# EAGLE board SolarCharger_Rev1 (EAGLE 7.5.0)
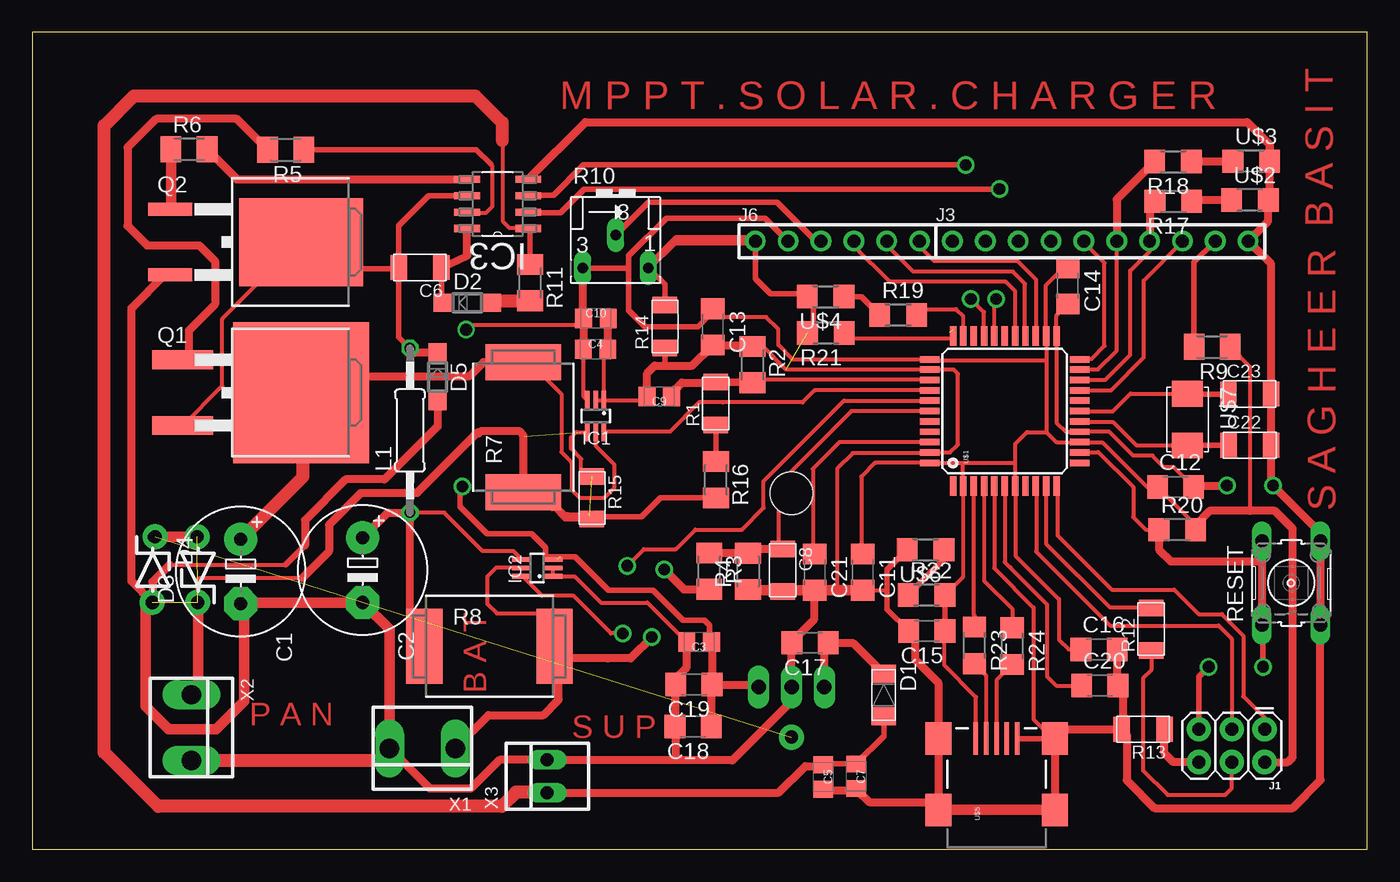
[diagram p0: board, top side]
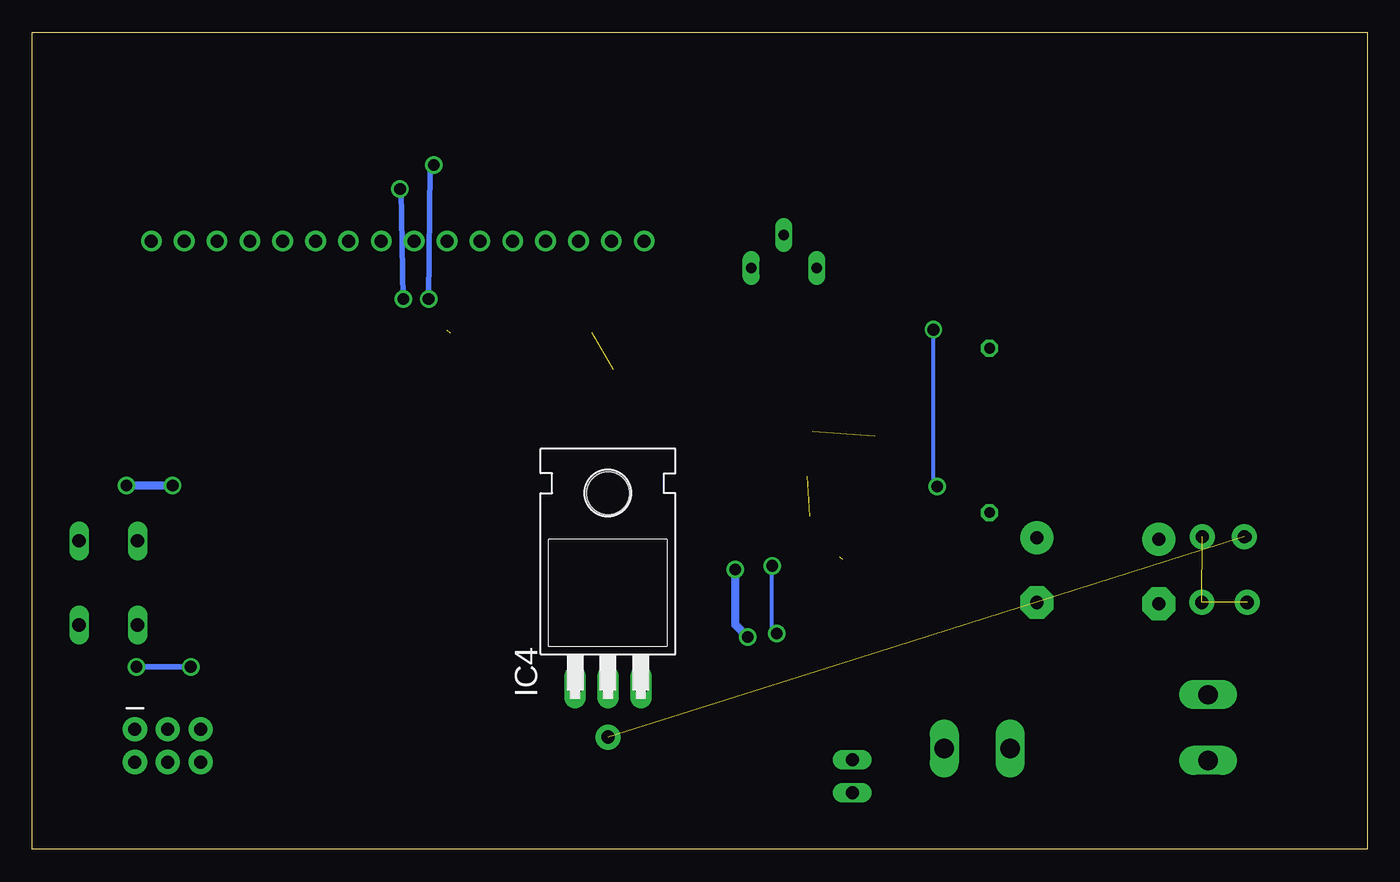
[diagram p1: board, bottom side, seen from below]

Size 103.17 x 63.12 mm. Coordinates in mm from the lower left corner, seen from the top.
Outline: 0,0 103.17,0 103.17,63.12 0,63.12 0,0
Copper layers (1*16): Top 0.035mm / dielectric 1.5mm / Bottom 0.035mm
Design rules "default": minimum track width 10mil, minimum drill 24mil, track to track 8mil, track to pad 8mil, pad to pad 8mil, via to via 8mil, smd to smd 8mil, copper to edge 40mil, drill to drill 8mil, minimum pad ring 10mil, minimum via ring 8mil, stop-mask expansion 4mil, vias tented up to drill 0mil, thermal gap 10mil

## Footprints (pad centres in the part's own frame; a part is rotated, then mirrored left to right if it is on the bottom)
10MM = drill 1.016 pad 2.54: + -2.5,0 | drill 1.016 pad 2.54 octagon: - 2.5,0
C0805 = smd 1.3 x 1.5: 1 -0.95,0; 2 0.95,0
C1206FAB = smd 1.27 x 1.905: 1 -1.651,0; 2 1.651,0
C1206 = smd 1.6 x 1.8: 1 -1.4,0; 2 1.4,0
MINI-SMA = smd 1.4 x 1.9: ANODE 1.65,0; KATHODE -1.65,0
SOD123 = smd 1.4 x 1.4: A 1.9,0; C -1.9,0
ZDIO-5 = drill 0.813 octagon: A 2.54,0; C -2.54,0
SC70-6_LONG = smd 0.35 x 1.5: 1 -0.65,-1.2; 2 0,-1.2; 3 0.65,-1.2; 4 0.65,1.2; 5 0,1.2; 6 -0.65,1.2
SOIC8 = smd 1.981 x 0.559: 1 -2.362,1.905; 2 -2.362,0.635; 3 -2.362,-0.635; 4 -2.362,-1.905; 5 2.362,-1.905; 6 2.362,-0.635; 7 2.362,0.635; 8 2.362,1.905
TO220H = drill 1.118 long: 1 -2.54,-10.16; 2 0,-10.16; 3 2.54,-10.16 | hole 3.302: 0,4.826
2X3 = drill 1.016 pad 1.88: 1 0,0; 2 0,2.54; 3 2.54,0; 4 2.54,2.54; 5 5.08,0; 6 5.08,2.54
100MIL_10X_ROUND = drill 1 pad 1.6: 1 -8.89,0; 2 -6.35,0; 3 -3.81,0; 4 -1.27,0; 5 1.27,0; 6 3.81,0; 7 6.35,0; 8 8.89,0; 9 11.43,0; 10 13.97,0
100MIL_6X_ROUND = drill 1 pad 1.6: 1 -6.35,0; 2 -3.81,0; 3 -1.27,0; 4 1.27,0; 5 3.81,0; 6 6.35,0
0207/12 = drill 0.813 octagon: 1 -6.35,0; 2 6.35,0
TO263-3 = smd 1.45 x 4.7: 1 -2.54,-5.65; 3 2.54,-5.65 | smd 10.9 x 10.5: TAB 0,3.5
TO263-3@1 = smd 1 x 3.4: 1 -2.54,-6.6; 3 2.54,-6.6 | smd 6.8 x 9.6: TAB 0,3.5
R1206FAB = smd 1.27 x 1.905: 1 -1.651,0; 2 1.651,0
M1206 = smd 1.6 x 2: 1 -1.4,0; 2 1.4,0
SMR = smd 2.8 x 5.8: 1 5.029,0; 2 -5.029,0
B25X = drill 0.813 long: A 2.54,-1.905; E -2.54,-1.905; S 0,0.635
R1206 = smd 1.6 x 1.803: 1 -1.422,0; 2 1.422,0
B3F-10XX = drill 1.016 long: 1 -3.251,2.261; 2 3.251,2.261; 3 -3.251,-2.261; 4 3.251,-2.261
SPARKFUN-DIGITALIC_TQFP44 = smd 1.5 x 0.5: 1 -5.8,4; 2 -5.8,3.2; 3 -5.8,2.4; 4 -5.8,1.6; 5 -5.8,0.8; 6 -5.8,0; 7 -5.8,-0.8; 8 -5.8,-1.6; 9 -5.8,-2.4; 10 -5.8,-3.2; 11 -5.8,-4; 23 5.8,-4; 24 5.8,-3.2; 25 5.8,-2.4; 26 5.8,-1.6; 27 5.8,-0.8; 28 5.8,0; 29 5.8,0.8; 30 5.8,1.6; 31 5.8,2.4; 32 5.8,3.2; 33 5.8,4 | smd 0.5 x 1.5: 12 -4,-5.8; 13 -3.2,-5.8; 14 -2.4,-5.8; 15 -1.6,-5.8; 16 -0.8,-5.8; 17 0,-5.8; 18 0.8,-5.8; 19 1.6,-5.8; 20 2.4,-5.8; 21 3.2,-5.8; 22 4,-5.8; 34 4,5.8; 35 3.2,5.8; 36 2.4,5.8; 37 1.6,5.8; 38 0.8,5.8; 39 0,5.8; 40 -0.8,5.8; 41 -1.6,5.8; 42 -2.4,5.8; 43 -3.2,5.8; 44 -4,5.8
LED1206 = smd 1.6 x 1.803: 1 -1.422,0; 2 1.422,0
USB_MINIB = smd 2.5 x 0.35: D+ 3.77,0; D- 3.77,0.8; GND 3.77,-1.6; ID 3.77,-0.8; VBUS 3.77,1.6 | smd 2.5 x 2: SHIELD@1 -1.73,-4.5; SHIELD@2 -1.73,4.5; SHIELD@3 3.77,4.5; SHIELD@4 3.77,-4.5
2-SMD-5X3MM = smd 2 x 2.4: P$1 -2,0; P$2 2,0
200MIL_2X = drill 1.5 long: 1 -2.54,0; 2 2.54,0
22-23-2021 = drill 1 long: 1 -1.27,0; 2 1.27,0

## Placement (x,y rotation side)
C1  680u  [10MM]  16.1,21.46 270 top
C2  820u  [10MM]  25.53,21.56 270 top
C3  100n  [C0805]  51.54,16 180 top
C4  100n  [C0805]  43.54,38.63 0 top
C5  100n  [C0805]  61.14,5.59 270 top
C6  100n  [C1206FAB]  29.97,44.94 180 top
C7  1u  [C0805]  63.68,5.64 270 top
C8  100n  [C1206FAB]  57.99,21.56 270 top
C9  100n  [C0805]  48.46,34.98 180 top
C10  100n  [C0805]  43.56,41.02 0 top
C11  0.1u  [C1206]  64.19,21.41 270 top
C12  0.1u  [C1206]  88.37,27.99 0 top
C13  0.1u  [C1206]  52.6,40.36 270 top
C14  0.1u  [C1206]  80.04,43.54 270 top
C15  0.1u  [C1206]  69.14,16.87 180 top
C16  0.1u  [C1206]  82.45,15.44 0 top
C17  470u  [C1206]  60.12,15.95 180 top
C18  1uf  [C1206]  51.08,9.47 180 top
C19  0.1u  [C1206]  51.13,12.73 180 top
C20  0.1u  [C1206]  82.5,12.65 0 top
C21  0.1u  [C1206]  60.48,21.41 270 top
C22  18pF  [C1206FAB]  94.11,31.22 0 top
C23  18pF  [C1206FAB]  94.1,35.17 0 top
D1  CDBM1100-G  [MINI-SMA]  65.81,11.91 270 top
D2  SCHOTTKYSOD123  [SOD123]  33.62,42.23 0 top
D3  15V  [ZDIO-5]  12.8,21.59 90 top
D4  5V  [ZDIO-5]  9.32,21.59 270 top
D5  SCHOTTKYSOD123  [SOD123]  31.33,36.5 270 top
IC1  INA213LONG  [SC70-6_LONG]  43.54,33.48 180 top
IC2  INA213LONG  [SC70-6_LONG]  39.01,21.74 90 top
IC3  IR2104  [SOIC8]  35.97,49.86 180 top
IC4  7805T  [TO220H]  58.68,22.69 0 bottom
J1  FEMALE 2x3  [2X3]  95.25,9.27 180 top
J3  Digital2  [100MIL_10X_ROUND]  80.01,46.99 0 top
J6  Analog  [100MIL_6X_ROUND]  62.23,46.99 0 top
L1  100u  [0207/12]  29.18,32.36 90 top
Q1  IPB136N08N3  [TO263-3]  17.27,35.28 270 top
Q2  IPB136N08N3  [TO263-3@1]  17.27,46.91 270 top
R1  6k  [R1206FAB]  52.83,34.44 90 top
R2  10k  [M1206]  55.68,37.44 270 top
R3  22k  [M1206]  52.32,21.49 270 top
R4  10k  [M1206]  55.32,21.46 90 top
R5  10  [M1206]  19.58,54.05 180 top
R6  10  [M1206]  12.12,54.08 0 top
R7  shunt 1  [SMR]  37.95,32.6 90 top
R8  shunt 2  [SMR]  35.33,15.69 0 top
R9  220  [M1206]  91.19,38.81 180 top
R10  10k  [B25X]  45.09,46.81 0 top
R11  10  [M1206]  38.48,43.77 270 top
R12  0  [R1206FAB]  86.48,17 90 top
R13  0  [R1206FAB]  85.85,9.27 180 top
R14  0  [R1206FAB]  48.9,40.39 90 top
R15  0  [R1206FAB]  43.26,27.15 270 top
R16  33k  [M1206]  52.83,28.55 270 top
R17  499  [R1206]  88.19,50.06 180 top
R18  499  [R1206]  88.16,53.14 180 top
R19  499  [R1206]  66.93,41.27 0 top
R20  10k  [R1206]  88.49,24.69 0 top
R21  680  [R1206]  61.34,39.9 180 top
R22  499  [R1206]  69.11,19.63 0 top
R23  22  [R1206]  72.82,15.75 270 top
R24  22  [R1206]  75.74,15.7 270 top
RESET  [B3F-10XX]  97.31,20.57 90 top
U$1  ATMEGA32U4TQFP  [SPARKFUN-DIGITALIC_TQFP44]  75.16,33.86 90 top
U$2  LED  [LED1206]  94.11,50.16 0 top
U$3  LED  [LED1206]  94.21,53.16 0 top
U$4  LED  [LED1206]  61.32,42.7 180 top
U$5  USB_MINIB  [USB_MINIB]  74.52,4.78 90 top
U$6  LED  [LED1206]  69.04,23.14 180 top
U$7  CRYSTAL  [2-SMD-5X3MM]  89.28,33.2 270 top
X1  Battery  [200MIL_2X]  30.15,7.8 180 top
X2  Pannel  [200MIL_2X]  12.29,9.4 270 top
X3  Supply  [22-23-2021]  39.8,5.64 90 top

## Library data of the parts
C1-C5 C7 C9 C10 = 00Capacitor
C6 C8 C22 C23 D1 R1 R12-R15 R17-R24 U$2-U$7 = fab
C11-C21 L1 R2-R6 R9 R11 R16 = rcl
D2 D5 = 00Diode
D3 D4 = diode
IC1 IC2 = 00Sensor; GAIN: 50
IC3 = 00Logic
IC4 = linear
J1 = SparkFun-Connectors; PROD_ID: CONN-11566
J3 J6 X1 X2 = 00Connector
Q1 Q2 = 00Mosfet
R7 R8 = resistor-shunt; OC_FARNELL: unknown; OC_NEWARK: unknown
R10 = pot
RESET = switch-omron; MPN: B3F-1000; OC_FARNELL: 176432; OC_NEWARK: 36M3542
U$1 = SparkFun-Retired; PROD_ID: IC-11161
X3 = 00Connector; MF: MOLEX; MPN: 22-23-2021; OC_FARNELL: 1462926; OC_NEWARK: 25C3832

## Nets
!SD!: IC3.3 U$1.30
+5V: C3.1 C4.1 C10.1 C11.1 C12.1 C13.1 C14.1 C15.1 C16.1 C18.1 C19.1 IC1.3 IC2.3 IC4.3 J1.2 J6.2 R9.1 R10.E R20.2 R22.2 U$1.2 U$1.7 U$1.14 U$1.24 U$1.34 U$1.44 U$5.VBUS
+12V: C5.1 C7.1 D1.ANODE IC3.1 R11.1 X3.1
AREF: C21.1 U$1.42
BATTERY: IC2.5 R3.2 R8.1 X1.1
D4: J3.5 U$1.22
D5: J3.6 R18.2 U$1.21
D6: J3.7 R17.2 U$1.20
D7: J3.8 U$1.19
D13: R19.2 U$1.32
D+: R24.1 U$1.4
D-: R23.1 U$1.3
E: J6.6 U$1.25
GND: C1.- C2.- C3.2 C4.2 C5.2 C7.2 C8.2 C9.2 C10.2 C11.2 C12.2 C13.2 C14.2 C15.2 C16.2 C17.2 C18.2 C19.2 C20.2 C21.2 C22.2 C23.2 D4.A D5.A IC1.1 IC1.2 IC2.1 IC2.2 IC3.4 IC4.2 J3.10 J6.1 Q2.3 R2.1 R4.1 R13.2 R14.1 R21.2 RESET.3 RESET.4 U$1.5 U$1.15 U$1.23 U$1.35 U$1.43 U$2.2 U$3.2 U$4.2 U$5.GND U$5.SHIELD@1 U$5.SHIELD@2 U$5.SHIELD@3 U$5.SHIELD@4 U$6.2 X1.2 X2.2 X3.2
IIN_SENSE: IC1.6 U$1.37
IOUT_SENSE: IC2.6 U$1.38
MISO: J1.1 U$1.11
MOSI: R12.2 U$1.10
N$1: J1.4 R12.1
N$2: J1.6 R13.1
N$3: R10.A R14.2
N$4: Q1.1 R5.2
N$5: R15.1 R16.2
N$7: Q2.1 R6.1
N$9: J3.9 R9.2
N$10: J6.3 R10.S
N$11: D2.A R11.2
N$12: C6.1 D2.C IC3.8
N$14: IC3.7 R5.1
N$15: IC3.5 R6.2
N$17: R1.1 R16.1
N$19: D3.A D4.C
N$20: C17.1 D1.KATHODE IC4.1
N$21: R17.1 U$2.1
N$22: R18.1 U$3.1
N$23: R19.1 U$4.1
N$24: R21.1 U$1.33
N$25: R24.2 U$5.D+
N$26: R22.1 U$6.1
N$27: R23.2 U$5.D-
PANNEL: D3.C IC1.4 R7.2 R15.2 X2.1
PWM: IC3.2 U$1.29
RESET: J1.5 R20.1 RESET.1 RESET.2 U$1.13
RS: J6.4 U$1.27
RW: J6.5 U$1.26
SCK: J1.3 U$1.9
SWITCHNODE: C6.2 D5.C IC3.6 L1.2 Q1.3 Q2.TAB
UCAP: C20.1 U$1.6
VIN: C1.+ IC1.5 Q1.TAB R7.1
VIN_SENSE: C9.1 R1.2 R2.2 U$1.36
VOUT: C2.+ IC2.4 L1.1 R8.2
VOUT_SENSE: C8.1 R3.1 R4.2 U$1.39
XTAL1: C23.1 U$1.17 U$7.P$1
XTAL2: C22.1 U$1.16 U$7.P$2

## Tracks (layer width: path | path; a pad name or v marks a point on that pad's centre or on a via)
!SD!  (via drill 0.9)
  Top 0.305: U$1.30 73.56,41.5 v72.54,42.52
  Top 0.406: IC3.3 38.38,50.55 40.28,50.55 42.62,52.88 v72.14,52.88
  Bottom 0.406: v72.14,52.88 72.42,52.6 v72.54,42.52
+5V  (via drill 0.9)  (1 unrouted)
  Top 0.305: U$1.7 75.97,28.05 | 86.97,28.02 C12.1 | U$5.VBUS 72.95,8.57 72.95,11.76 70.51,14.2 70.51,16.79 70.1,17.2 C15.1 | C14.1 79.71,44.94 78.36,43.59 U$1.24 78.38,39.63 78.38,37.8 | 78.38,37.8 78.38,32.23 | 78.38,32.23 79.16,31.46 U$1.14 80.97,31.45 82.7,31.45 86.16,27.99 C12.1 | 75.97,28.05 76,28.02 76,22.68 79.35,19.33 79.35,16.2 80.11,15.44 C16.1 | 75.97,28.05 75.97,29.84 | 75.97,29.84 75.97,31.32 76.89,32.23 78.38,32.23 | 78.38,37.8 69.42,37.8 U$1.34 58.76,37.86 57.66,38.96 57.66,40.18 56.72,41.12 53.24,41.12 C13.1 53.19,42.09 | U$1.44 69.37,29.84 71.93,29.84 | 71.93,29.84 75.97,29.84 | 71.93,29.84 71.93,28.08 U$1.2 71.96,21.06 R22.2 | C11.1 64.19,23.47 64.08,23.58 64.08,28.8 65.13,29.85 U$1.44 | U$1.44 | 52.4,16.09 C3.1 | 40.55,22.39 IC2.3 40.57,22.39 40.56,22.4 40.57,22.4 | 40.77,22.61 40.77,22.59 40.77,22.61 | v33.53,40.15 33.9,40.52 42.61,40.52 | IC1.3 42.61,34.95 42.61,39.13 | C12.1 89.92,25.04 | R9.1 94.12,37.28 94.12,26.14
  Top 0.406: R22.2 C15.1 | J6.2 56.64,48.77 49.02,48.77 46.1,45.85 46.1,44.96 | 46.1,44.96 46.1,41.66 47.37,40.39 51.44,40.39 52.6,41.55 C13.1 | R10.E 46.05,44.91 46.1,44.96 | C3.1 52.34,16.15 52.34,17.31 51.96,17.69 50.31,17.69 47.98,20.02 44.53,20.02 41.94,22.61 40.77,22.61 | 40.77,22.59 39.66,22.59 39.66,23.31 38.6,24.38 35.16,24.38 33.08,26.46 33.08,27.86 v33.23,28.02
  Top 0.61: R10.E 42.55,41.09 C10.1 42.61,40.52 42.61,39.13 42.61,38.66 C4.1 | R20.2 89.92,25.04 91.01,26.14 94.12,26.14 96.04,26.14 97.41,24.77 97.41,7.11 97.03,6.73 J1.2 | C3.1 52.53,16 C19.1 | C18.1 52.48,12.68 C19.1 | C19.1 55.95,12.72 IC4.3
  Bottom 0.305: v33.23,28.02 33.53,28.32 v33.53,40.15
+12V
  Top 0.305: IC3.1 38.29,47.99 36.88,47.99 36.4,48.48 36.4,54.69
  Top 0.406: C5.1 61.19,6.59 C7.1 65.81,8.72 D1.ANODE | 36.32,54.76 36.4,54.69 | IC3.1 38.48,47.8 R11.1
  Top 0.61: 61.08,6.48 C5.1 61.03,6.43 59.74,6.43 57.68,4.37 X3.1
  Top 1.016: X3.1 39.75,4.42 37.39,4.42 36.27,3.3 9.73,3.3 5.54,7.49 5.54,55.91 7.85,58.22 34.24,58.22 36.32,56.13 36.32,54.76
AREF
  Top 0.305: 60.5,22.84 C21.1 60.34,22.95 60.34,29.4 62.4,31.46 U$1.42
BATTERY  (via drill 0.9)
  Top 0.305: IC2.5 37.8,21.75 35.85,21.75 35.16,21.07 35.16,18.96 35.91,18.22 41.01,18.22
  Top 0.61: v47.89,16.39 46.25,14.75 44.47,14.75 40.68,14.75 | 41.01,18.22 40.34,18.22 40.34,15.72 R8.1 40.36,15.07 40.68,14.75 | X1.1 35.26,10.37 39.5,10.37 40.68,11.55 40.68,14.75 | v48.83,21.62 50.37,20.09 R3.2
  Bottom 0.61: v47.89,16.39 48.83,17.33 v48.83,21.62
D4
  Top 0.305: U$1.22 81,37.9 81.89,37.9 82.88,38.89 82.88,45.31 81.28,46.91 J3.5
D5
  Top 0.305: U$1.21 80.98,37.08 82.37,37.08 83.82,38.53 J3.6
  Top 0.61: R18.2 83.82,50.22 J3.6
D6
  Top 0.305: U$1.20 80.97,36.27 82.93,36.27 84.86,38.2 84.86,44.7 86.36,46.2 J3.7
  Top 0.61: R17.2 86.36,49.66 J3.7
D7
  Top 0.305: U$1.19 80.98,35.48 83.39,35.48 85.9,38 85.9,43.94 88.9,46.94 J3.8
D13
  Top 0.305: U$1.32 71.96,41.17 71.4,41.73 68.89,41.73 68.43,41.27 R19.2
D+
  Top 0.305: U$1.4 73.56,20.75 75.74,18.57 R24.1
D-
  Top 0.305: U$1.3 72.75,28.05 72.75,18.14 72.82,18.06 R23.1
E
  Top 0.305: U$1.25 77.56,44.06 76.17,45.44 69.72,45.44 68.58,46.58 J6.6
GND  (via drill 0.9)  (1 unrouted)
  Top 0.305: U$1.43 | U$1.43 70.94,30.66 71.55,31.27 71.55,36.73 71.22,37.06 U$1.35 58.27,37.06 56.47,38.86 R2.1 | C12.2 88.24,29.52 87.48,29.52 86.59,30.4 85.09,30.4 83.24,32.26 U$1.15 79.88,32.26 79.17,32.97 79.17,39.65 U$1.23 79.16,41.26 C14.2 | U$1.5 74.35,28.05 74.35,21.72 77.39,18.67 77.39,10.03 78.88,8.54 U$5.SHIELD@4 | C11.2 66.04,20.01 66.06,20.04 | C21.2 61.74,20.01 | U$1.43 69.31,30.61 63.42,30.61 62.21,29.4 62.21,20.17 62.37,20.01 | IC1.2 IC1.1 | IC1.1 47.22,34.68 C9.2 | IC1.1 44.19,38.33 C4.2 | C3.2 47.54,19.05 43.94,19.05 41.9,21.09 IC2.1 IC2.2 | 9.3,20.69 9.3,20.65 | 10.6,21.99 19.6,21.99 | U$4.2 60.1,42.49 60.38,42.49
  Top 0.406: U$5.GND U$5.SHIELD@4 | U$5.SHIELD@3 70,8.52 70,2.95 | C12.2 89.87,28.09 | U$6.2 66.06,21.59 66.06,20.04 66.06,18.54 C15.2 | U$6.2 | C7.2 63.63,4.64 C5.2 | 16.2,19.07 16.33,18.94 | C10.2 44.51,38.8 44.45,38.73 | R14.1 48.9,37.49 48.77,37.36 | J6.1 55.88,44.09 57.05,42.93 59.66,42.93 U$4.2 | 60.38,42.49 60.38,40.35 R21.2 | 21.08,23.47 19.6,21.99
  Top 0.61: U$3.2 95.63,50.27 U$2.2 95.53,48.54 J3.10 95.75,45.22 C23.2 95.75,31.23 C22.2 95.76,28.25 v95.91,28.09 99.57,24.43 RESET.4 RESET.3 99.57,5.33 97.41,3.17 86.74,3.17 84.58,5.33 84.58,8.87 84.3,9.14 R13.2 | U$5.SHIELD@4 U$5.SHIELD@1 | 70.02,3.63 U$5.SHIELD@3 70.02,12.88 68.22,14.68 68.22,16.38 C15.2 | 70.02,3.63 U$5.SHIELD@2 | C5.2 61.2,4.57 63.75,4.57 64.69,3.63 70.02,3.63 | 49.68,10.01 49.68,12.68 C19.2 49.48,12.97 50.59,14.08 C3.2 50.33,15.75 | 49.68,10.01 C18.2 49.73,9.42 | U$5.SHIELD@4 79.25,8.77 79.25,8.76 79.76,9.27 R13.2 | C4.2 44.49,41 C10.2 | C9.2 47.51,36.77 48.11,37.36 48.77,37.36 51.01,37.36 C13.2 56.37,38.96 R2.1 | 49.68,10.01 49.73,9.95 49.73,6.96 49.68,6.91 49.71,6.88 49.73,6.91 X3.2 | X3.2 36.12,6.91 33.88,4.67 30.73,4.67 X1.2 | Q2.3 10.24,44.37 7.67,41.81 7.67,20.7 D4.A 9.32,20.63 9.3,20.65 | IC3.4 42.74,56.18 93.89,56.18 95.63,54.44 U$3.2 | 95.63,54.15 U$3.2 | 89.87,28.09 v92.33,28.09 | 83.92,15.52 C16.2 83.85,12.7 C20.2 83.9,12.49 84.33,12.06 84.33,9.37 R13.2 | 78.99,9.14 79.02,9.11 U$5.SHIELD@4 | D5.A 31.33,32.68 27.23,28.57 24.23,28.57 21.08,25.43 21.08,23.47 | C8.2 58.1,20.01 C21.2 60.45,19.99 60.45,17.78 58.72,16.05 C17.2 58.68,15.91 IC4.2 58.68,11.19 58.67,11.18 58.42,11.18 54.1,6.86 39.85,6.86 X3.2 | 9.3,20.69 10.6,21.99
  Top 0.813: 70,2.95 70.1,3.04 U$5.SHIELD@1 | C11.2 62.37,20.01 C21.2 55.37,20.01 R4.1 | X1.2 27.61,16.98 C2.- 16.2,19.07 C1.- | 16.33,18.94 16.38,18.89 16.38,11.43 14.22,9.27 10.54,9.27 8.76,11.05 8.76,18.92 8.89,19.05 D4.A
  Top 1.016: X2.2 26.67,6.86 X1.2
  Bottom 0.61: v92.33,28.09 v95.91,28.09
IIN_SENSE
  Top 0.305: U$1.37 60.46,35.45 59.53,34.52 53.38,34.52 53.37,34.52 51.54,34.52 49.29,32.28 IC1.6
IOUT_SENSE  (via drill 0.9)
  Top 0.305: v45.63,16.66 45.62,16.68 44.73,16.68 41.82,19.58 39.39,19.58 37.88,21.09 IC2.6 | v45.99,21.9 47.27,23.18 49.74,23.18 51.24,24.69 54.84,24.69 56.53,26.38 56.53,28.44 62.75,34.66 U$1.38
  Bottom 0.305: v45.63,16.66 45.99,17.01 v45.99,21.9
MISO
  Top 0.305: J1.1 95.25,10.16 93.6,11.81 93.6,16.51 91.95,18.16 90.17,18.16 88.27,20.07 83.44,20.07 79.25,24.26 79.25,27.97 U$1.11
MOSI
  Top 0.305: U$1.10 | U$1.10 78.36,23.62 83.29,18.69 86.44,18.69 R12.2
N$1
  Top 0.305: R12.1 86.49,15.72 86.49,13.84 85.85,13.21 85.85,6.1 87.76,4.19 92.2,4.19 92.71,4.7 J1.4
N$2
  Top 0.61: J1.6 88.21,6.73 87.52,7.42 87.52,9.26 R13.1
N$3
  Top 0.406: R14.2 48.9,43.64 47.75,44.78 47.75,44.96 49.66,46.86 56.01,46.86 55.63,47.24 49.78,47.24 47.62,45.09 R10.A
N$4
  Top 0.305: 12.09,38.08 11.88,38.08 Q1.1
  Top 0.61: R5.2 15.8,56.44 9.58,56.44 7.37,54.23 7.37,48.16 8.87,46.66 12.9,46.66 14.12,45.44 14.12,42.11 12.09,40.08 12.09,38.08
N$5  (1 unrouted)
  Top 0.305: R15.1 42.73,29.1 42.62,29.1 42.43,28.91 42.43,30.16 41.62,30.97 41.62,31.8 42.04,32.22 42.82,32.22
  Top 0.406: R16.2 48.56,27.15 47.09,25.68 43.1,25.68 43.05,25.73 43.05,25.6 43,25.55 41.17,25.55 40.39,26.34 40.18,26.34 38.86,27.66
N$7
  Top 0.813: Q2.1 10.72,49.5 R6.1
N$9
  Top 0.406: J3.9 89.79,45.34 R9.2
N$10
  Top 0.406: R10.S 47.62,49.99 57.56,49.99 60.55,46.99 J6.3
N$11
  Top 1.016: D2.A 35.55,42.37 R11.2
N$12
  Top 0.406: 31.72,42.31 31.62,42.41 C6.1
  Top 0.61: D2.C 31.72,42.31 | C6.1 33.6,45.86 IC3.8
N$14
  Top 0.305: 33.66,49.17 35.06,49.17 35.57,49.69 35.57,52.78 35.44,52.91
  Top 0.406: IC3.7 33.66,49.17 | R5.1 34.3,54.05 35.44,52.91
N$15
  Top 0.61: R6.2 15.83,51.77 IC3.5
N$17
  Top 0.406: 53.37,29.95 52.93,29.95 52.86,30.02 52.86,32.77 R1.1
  Top 0.61: 53.37,29.95 R16.1
N$19
  Top 0.813: D3.A D4.C
N$20
  Top 0.61: IC4.1 61.22,15.15 C17.1 63.42,15.95 D1.KATHODE
N$21
  Top 0.61: R17.1 89.71,50.16 U$2.1
N$22
  Top 0.61: R18.1 89.61,53.16 U$3.1
N$23
  Top 0.406: U$4.1 64.08,42.7 R19.1
N$24  (1 unrouted)
  Top 0.305: 71.22,40.23 71.25,40.26 71.25,39.75 U$1.33 | 71.16,40.16 U$1.33 | R21.1 62.76,39.7 62.97,39.5 71,39.5 U$1.33
N$25
  Top 0.305: R24.2 74.52,13.06 U$5.D+
N$26
  Top 0.406: U$6.1 70.46,22.4 R22.1
N$27
  Top 0.305: R23.2 73.72,13.42 U$5.D-
N$28  (via drill 1.02 pad 1.93)  (1 unrouted)
  other vias: 9.48,24.14 58.68,8.67
N$29  (via drill 1.02 pad 1.93)  (2 unrouted)
  other vias: 12.75,24.14 9.28,19.07 12.78,19.07
PANNEL  (1 unrouted)
  Top 0.305: R7.2 39.12,26.4 40.7,26.4 41.37,25.73 | 37.95,31.99 38.03,31.9 38.03,27.94 | 20.86,20.95 12.94,20.95 12.8,20.82
  Top 0.406: 34.49,32.13 34.42,32.21 | 12.8,20.82 D3.C
  Top 0.61: 34.42,32.21 29.74,27.53 25.4,27.53 22.93,25.06 22.93,23.02 20.86,20.95 | 34.49,32.13 34.69,32.33 37.61,32.33 37.95,31.99 R7.2 | 41.37,25.73 43.03,25.73 R15.2
  Top 0.813: X2.1 12.8,12.45 D3.C
PWM  (via drill 0.9)
  Top 0.305: U$1.29 74.36,42.38 v74.5,42.52
  Top 0.406: IC3.2 38.38,49.17 40.82,49.17 42.65,51 v74.75,51
  Bottom 0.406: v74.75,51 74.68,50.93 v74.5,42.52
RESET  (via drill 0.9)
  Top 0.305: U$1.13 | U$1.13 80.98,30.68 82.4,30.68 85.09,27.99 85.09,25.65 86.06,24.69 R20.1
  Top 0.406: RESET.1 95.12,17.25 v95.12,14.1 | v90.93,14.1 90.17,13.34 J1.5
  Top 0.61: 94.56,23.82 RESET.2 95.05,22.24 | 95.05,22.24 RESET.1 | R20.1 87.08,24.68 87.08,23.16 87.99,22.24 95.05,22.24
  Bottom 0.406: v95.12,14.1 v90.93,14.1
RS
  Top 0.305: U$1.27 75.97,39.67 75.97,43.1 75.23,43.84 66.27,43.84 63.5,46.61 J6.4
RW
  Top 0.305: U$1.26 76.73,39.68 76.73,43.69 75.79,44.63 68.1,44.63 66.04,46.69 J6.5
SCK
  Top 0.305: U$1.9 77.6,28.02 77.6,22.99 83.31,17.27 91.69,17.27 92.71,16.26 J1.3 92.71,9.53
SWITCHNODE
  Top 0.305: Q1.3 14.69,35.8 14.69,40.98 17.89,44.18 | 17.89,44.18 18.15,44.45 18.15,45.17 | 18.8,44.53 18.81,44.54 19.6,44.54 19.55,44.59 19.55,46.21 17.89,44.55 17.89,44.18
  Top 0.406: IC3.6 30.64,50.51 28.32,48.19 C6.2 | C6.2 28.21,44.84 23.05,44.84 22.68,44.46 20.77,44.46 | L1.2 28.32,39.58 C6.2
  Top 0.61: 17.98,44.17 18.44,44.17 18.8,44.53 19.48,45.21 19.48,46.38 19.96,46.86 21.29,46.86 21.23,46.91 Q2.TAB | 29.55,38.35 L1.2 29.49,38.4 D5.C
  Top 0.813: 20.75,44.04 20.77,44.06 20.77,44.46 Q2.TAB
UCAP
  Top 0.305: U$1.6 75.18,28.03 75.16,28.01 75.16,22.2 75.18,22.17 75.6,21.75 78.44,18.92 78.44,13.36 79.15,12.65 C20.1
VIN
  Top 0.305: 43.56,32.25 IC1.5 43.54,31.17 44.98,29.72 44.98,27.93 44.23,27.17 42.28,27.17 41.68,27.78 41.68,29.9 40.89,30.68 40.89,35.17 39.49,36.58 39.93,36.58 40.58,37.23 38.35,37.23 R7.1
  Top 0.61: 20.93,28.79 20.93,34.01 23.48,36.56 33.79,36.56 34.87,37.63 R7.1
  Top 1.016: C1.+ 20.93,28.79 20.93,35.84 21.41,35.36 21.41,34.77 20.9,35.28 Q1.TAB
VIN_SENSE
  Top 0.305: U$1.36 56.56,36.26 R2.2
  Top 0.61: 56.19,35.89 R2.2 56.38,36.14 R1.2 53.27,36.05 50.2,36.05 49.41,35.27 C9.1
VOUT
  Top 0.305: IC2.4 37.18,23.02 36.77,23.02 36.76,23.03 34.82,23.03 31.84,26.01 L1.1
  Top 0.61: C2.+ 27.47,26.01 L1.1 29.18,16.81 R8.2
VOUT_SENSE
  Top 0.305: 58.14,23.2 C8.1 57.66,23.07 57.66,28.22 63.3,33.86 U$1.39
  Top 0.61: R4.2 52.35,22.86 R3.1 | 55.35,22.9 55.66,23.21 C8.1
  Top 0.813: R4.2 55.35,22.9
XTAL1
  Top 0.305: U$1.17 80.98,33.83 83.52,33.83 84.88,35.2 U$7.P$1
  Top 0.406: U$7.P$1 89.33,35.17 C23.1
XTAL2
  Top 0.305: U$1.16 81,33.02 83.52,33.02 85.34,31.2 U$7.P$2
  Top 0.406: U$7.P$2 89.3,31.22 C22.1

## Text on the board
Top: B A S I T | M P P T . S O L A R . C H A R G E R | S A G H E E R | B A T | P A N | S U P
